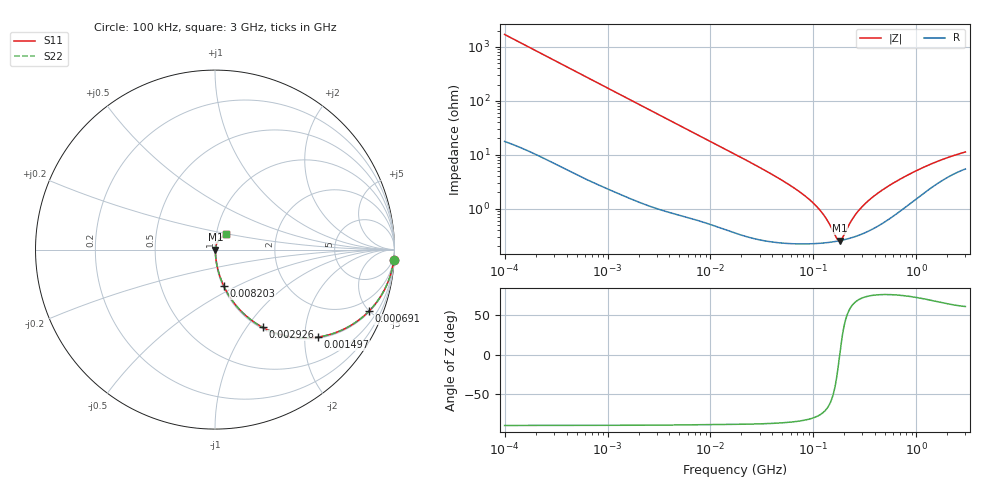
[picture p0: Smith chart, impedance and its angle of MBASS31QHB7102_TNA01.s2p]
! MBASS31QHB7102_TNA01  S-PARAMETER MODEL  ( Standard Model )
! Model Generated by TAIYO YUDEN Corporation (http://www.ty-top.com)
! Version 1.0
! TAIYO YUDEN Control No. 220601
! Copyright(c) 2013 TAIYO YUDEN CO.,LTD. All Rights Reserved.
! Product Description (link to TY-COMPAS)
! https://ds.yuden.co.jp/TYCOMPAS/or/detail?pn=MBASS31QHB7102KTNA01&u=M
! Products Name : Multilayer Ceramic Capacitors
! Characteristics :
!  Capacitance : 1000 [pF] , Rated Voltage : 630 [V] , TCC : X7R
!  Case Size : 3.2 x 1.6 / 0.126 x 0.063 [mm/inch] , Thickness : 1.15 / 0.045 [mm/inch]
!  (Conditions: Temperature = 25 [degC] , DC Bias Voltage = 0 [V])
! External Node Assignments :
!  1  o---| |---o  2
! GND o---------o GND
! Frequency Range : 100kHz  -  3GHz  [ 401 STEP ]
# MHZ S RI R 50
! Freq[MHz].  S11 Real  S11 Imag  S21 Real  S21 Imag  S12 Real  S12 Imag  S22 Real  S22 Imag
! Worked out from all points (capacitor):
!   401 points, 100 kHz to 3 GHz, reference 50 ohm
!   read as one part in series: C = 936 pF near 105.3 kHz
!   lowest |Z| = 254 mohm at 180.8 MHz (marker M1)
!   series resonance near 180.2 MHz, so ESL is about 830 pH
!   S11 on the Smith chart (normalised r, x): 100 kHz: 1, -34; 691 kHz: 1.06, -4.99; 1.497 MHz: 1.03, -2.31; 2.926 MHz: 1.02, -1.19; 8.203 MHz: 1.01, -0.43; 3 GHz: 1.11, +0.20
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0.1  0.9959 -0.0587  0.00407 0.0587  0.00407 0.0587  0.9959 -0.0587
0.252895  0.9769 -0.1443  0.0231 0.1443  0.0231 0.1443  0.9769 -0.1443
0.562235  0.9005 -0.2932  0.0995 0.2932  0.0995 0.2932  0.9005 -0.2932
0.690972  0.8582 -0.3425  0.1418 0.3425  0.1418 0.3425  0.8582 -0.3425
1.497078  0.5714 -0.4877  0.4286 0.4877  0.4286 0.4877  0.5714 -0.4877
2.925885  0.2649 -0.4328  0.7351 0.4328  0.7351 0.4328  0.2649 -0.4328
3.161081  0.2368 -0.4164  0.7632 0.4164  0.7632 0.4164  0.2368 -0.4164
4.899066  0.1181 -0.3122  0.8819 0.3122  0.8819 0.3122  0.1181 -0.3122
8.202936  0.0488 -0.2026  0.9512 0.2026  0.9512 0.2026  0.0488 -0.2026
17.7727  0.0131 -0.0976  0.9869 0.0976  0.9869 0.0976  0.0131 -0.0976
53.83243  0.00317 -0.0302  0.9968 0.0302  0.9968 0.0302  0.00317 -0.0302
97.38194  0.00239 -0.013  0.9976 0.013  0.9976 0.013  0.00239 -0.013
126.0104  0.00235 -0.00723  0.9977 0.00723  0.9977 0.00723  0.00235 -0.00723
167.3121  0.00247 -0.00147  0.9975 0.00147  0.9975 0.00147  0.00247 -0.00147
180.7614  0.00253 5.67e-05  0.9975 -5.67e-05  0.9975 -5.67e-05  0.00253 5.67e-05
195.2919  0.00261 0.00158  0.9974 -0.00158  0.9974 -0.00158  0.00261 0.00158
246.2744  0.00299 0.00623  0.997 -0.00623  0.997 -0.00623  0.00299 0.00623
287.4592  0.00337 0.00948  0.9966 -0.00948  0.9966 -0.00948  0.00337 0.00948
381.6779  0.00446 0.016  0.9955 -0.016  0.9955 -0.016  0.00446 0.016
547.5153  0.00705 0.0257  0.993 -0.0257  0.993 -0.0257  0.00705 0.0257
1281.618  0.0243 0.0562  0.9757 -0.0562  0.9757 -0.0562  0.0243 0.0562
3000  0.0596 0.0876  0.9404 -0.0876  0.9404 -0.0876  0.0596 0.0876
